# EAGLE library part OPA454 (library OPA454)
TexasInstruments High-Voltage (100V), High-Current (50mA) Operatioanl Amplifier, G = 1 Stable http://focus.ti.com/lit/ds/symlink/opa454.pdf
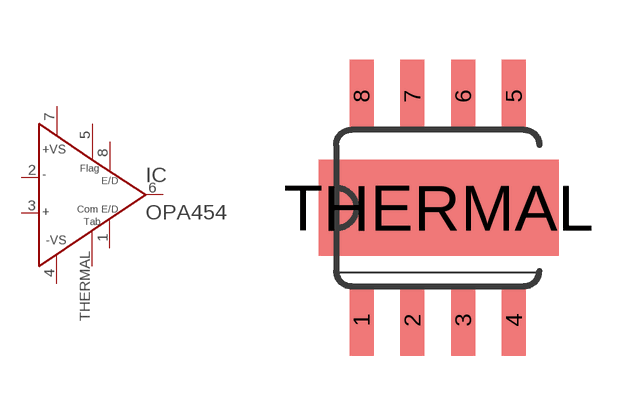
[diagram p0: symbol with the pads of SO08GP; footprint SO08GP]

Designator prefix IC

## OPA454 (Availability: Unavailable; Description: High Voltage _100V_ High-Current _50mA_ Operational Amplifiers G=1 Stable; MF: Texas Instruments; MP: OPA454; Package: None; Price: None)  [SO08GP]
1  E/DCOM  pas
2  IN-  in
3  IN+  in
4  -VS  pas
5  STATUS  pas
6  OUT  out
7  +VS  pas
8  E/D  pas
THERMAL  E/DCOM1  pas

## Footprint SO08GP (pad centres in mm)
smd 0.6 x 1.8: 1 -1.925,-2.8; 2 -0.655,-2.8; 3 0.615,-2.8; 4 1.885,-2.8; 5 1.885,2.8; 6 0.615,2.8; 7 -0.655,2.8; 8 -1.925,2.8
smd 6 x 2.4: THERMAL 0,0

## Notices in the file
This work is licensed under a Creative Commons Attribution-ShareAlike 4.0 International License (CC BY-SA) with Design Exception 1.0
